{attribute 'no_assign'}
FUNCTION_BLOCK FB_DO_IED_MUnn_LPHD1_PhyNam EXTENDS FB_AcsiCommonDataClass
VAR_INPUT
	vendor: FB_AcsiDATypeVisString255 := (Fc:=ACSI_FC_DC, sValue:='BECKHOFF', bLinkResult:=THIS^.AddDataToContainer(ipData:=vendor));
END_VAR
VAR
END_VAR

END_FUNCTION_BLOCK
